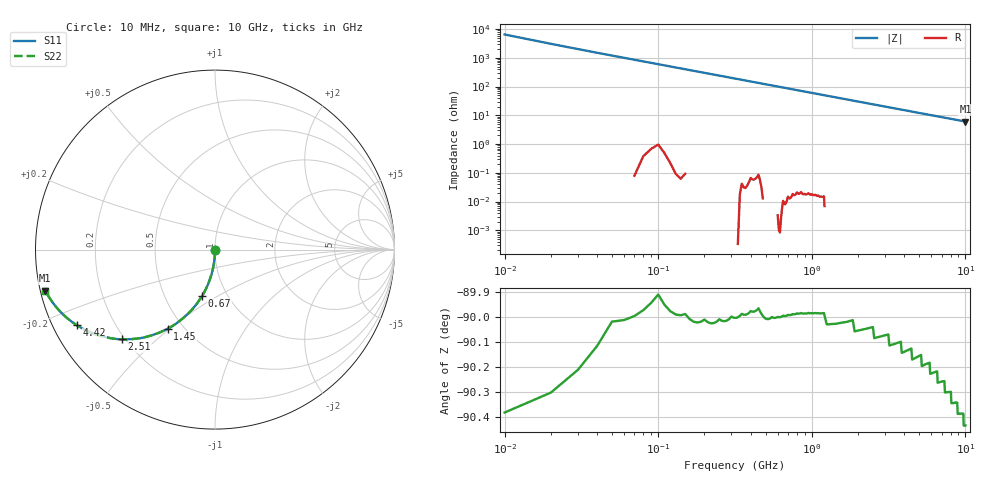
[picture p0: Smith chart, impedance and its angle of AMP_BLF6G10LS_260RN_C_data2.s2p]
! Created Mon Mar 29 11:12:16 2010
# ghz S ma R 50
! 2 Port Network Data from SP1.SP block
! freq  magS11  angS11  magS21  angS21  magS12  angS12  magS22  angS22
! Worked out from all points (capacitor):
!   1000 points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, 10 MHz to 10 GHz, reference 50 ohm
!   read as one part in shunt: C = 2.64 pF near 60 MHz
!   lowest |Z| = 6.09 ohm at 10 GHz (marker M1)
!   S11 on the Smith chart (normalised r, x): 10 MHz: 1.00, -0.01; 670 MHz: 0.76, -0.42; 1.45 GHz: 0.41, -0.49; 2.51 GHz: 0.19, -0.39; 4.42 GHz: 0.07, -0.25; 10 GHz: 0.01, -0.12
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0.01  0.003839 -89.8  1 -0.2  1 -0.2  0.003823 -89.7
0.04  0.01655 -90.8  0.9999 -1.0  0.9999 -1.0  0.01662 -90.8
0.07  0.02897 -91.6  0.9996 -1.7  0.9996 -1.7  0.0291 -91.6
0.09  0.03719 -92.2  0.9993 -2.1  0.9993 -2.1  0.03735 -92.2
0.13  0.05366 -93.1  0.9985 -3.1  0.9985 -3.1  0.05389 -93.1
0.19  0.07819 -94.5  0.9969 -4.5  0.9969 -4.5  0.07852 -94.5
0.27  0.1107 -96.4  0.9938 -6.4  0.9938 -6.4  0.1112 -96.3
0.38  0.1548 -99.0  0.9878 -9.0  0.9878 -9.0  0.1555 -98.9
0.52  0.211 -102.1  0.9775 -12.2  0.9775 -12.2  0.2103 -102.2
0.67  0.2676 -105.5  0.9635 -15.5  0.9635 -15.5  0.2672 -105.5
0.83  0.3249 -109.0  0.9456 -19.0  0.9456 -19.0  0.3248 -109.0
1.01  0.3853 -112.7  0.9225 -22.7  0.9225 -22.7  0.3855 -112.7
1.45  0.5145 -120.9  0.8576 -31.0  0.8576 -31.0  0.5142 -120.9
1.68  0.5704 -124.8  0.8212 -34.8  0.8212 -34.8  0.5706 -124.8
2.04  0.6452 -130.1  0.7644 -40.2  0.7644 -40.2  0.6448 -130.1
2.51  0.72 -136.1  0.694 -46.1  0.694 -46.1  0.7201 -136.1
3.34  0.8104 -144.1  0.5869 -54.2  0.5869 -54.2  0.81 -144.1
4.42  0.8773 -151.3  0.4807 -61.4  0.4807 -61.4  0.8774 -151.3
5.01  0.9007 -154.2  0.4356 -64.4  0.4356 -64.4  0.9007 -154.2
6.67  0.9407 -160.0  0.342 -70.3  0.342 -70.3  0.9403 -160.0
8.34  0.961 -163.8  0.28 -74.1  0.28 -74.1  0.9607 -163.8
10  0.9725 -166.4  0.2367 -76.8  0.2367 -76.8  0.9724 -166.3
